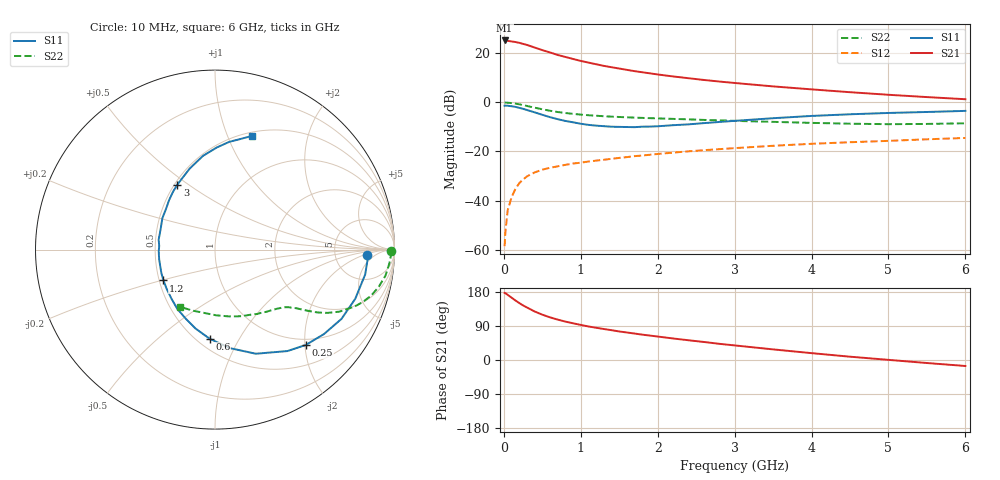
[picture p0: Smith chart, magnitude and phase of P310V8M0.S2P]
! SIEMENS Small Signal Semiconductors
! BFP181
! Si NPN RF Bipolar Junction Transistor in SOT143
! VCE = 10 V  IC = 8 mA
! Common Emitter S-Parameters:  March  1996
# GHz  S  MA  R  50
!  f  S11  S21  S12  S22
! GHz  MAG  ANG  MAG  ANG  MAG  ANG  MAG  ANG
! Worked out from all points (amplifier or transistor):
!   36 points, 10 MHz to 6 GHz, reference 50 ohm
!   highest |S21| = 25.1 dB at 10 MHz (marker M1)
!   |S21| within 3 dB of that: start of sweep to 413 MHz
!   unconditionally stable (mu >= 1): 1.558 GHz to end of sweep
!   at 250 MHz: K = 0.27, MSG = 27.5 dB, |S12| = -31.3 dB
!   at 1.4 GHz: K = 0.96, MSG = 18.6 dB, |S12| = -23.0 dB
!   at 6 GHz: K = 1.05, MAG = 6.5 dB, |S12| = -14.5 dB
!   S11 on the Smith chart (normalised r, x): 10 MHz: 12, -2; 250 MHz: 0.88, -2.02; 600 MHz: 0.58, -0.76; 1.2 GHz: 0.53, -0.20; 3 GHz: 0.52, +0.45; 6 GHz: 0.54, +1.23
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0.01  0.8483 -2.0  17.89 177.1  0.0012 73.8  0.9797 -0.6
0.02  0.852 -3.7  17.85 176.4  0.0023 85.7  0.9817 -1.6
0.05  0.8481 -9.4  17.55 171.9  0.0064 87.4  0.9749 -4.4
0.15  0.8036 -28.7  16.63 157.2  0.0174 73.2  0.9357 -12.8
0.2  0.7681 -37.8  16.03 150.4  0.0227 70.7  0.9072 -16.4
0.25  0.7336 -46.4  15.24 144.0  0.0271 66.5  0.8727 -19.6
0.3  0.6945 -54.5  14.53 138.6  0.0312 63.3  0.8386 -22.3
0.4  0.6231 -68.6  12.87 128.1  0.0376 57.9  0.7747 -26.5
0.5  0.5552 -81.4  11.38 119.6  0.0428 53.5  0.7183 -29.4
0.6  0.4971 -93.5  10.22 112.6  0.0467 51.4  0.6703 -31.5
0.7  0.4528 -103.9  9.089 106.6  0.05 49.7  0.6325 -32.9
0.8  0.4165 -113.4  8.278 101.3  0.0536 48.5  0.6032 -34.0
1.1  0.3468 -141.0  6.366 88.5  0.0626 46.1  0.5438 -36.6
1.2  0.3346 -149.1  5.886 85.1  0.0653 45.7  0.5314 -37.4
1.5  0.3157 -170.4  4.819 75.3  0.0741 45.1  0.5009 -39.9
1.8  0.3188 169.9  4.048 66.9  0.0828 43.9  0.4803 -43.1
2.2  0.3415 149.2  3.33 56.8  0.0948 42.1  0.4585 -47.9
3  0.4182 120.2  2.455 38.5  0.117 36.9  0.4181 -59.6
3.5  0.4732 107.3  2.092 28.0  0.1305 33.2  0.3993 -68.4
4.5  0.5686 89.1  1.595 8.7  0.1542 25.5  0.3664 -88.8
5.5  0.6332 76.9  1.27 -8.0  0.1768 18.8  0.3624 -110.5
6  0.6665 71.9  1.149 -15.8  0.1881 14.9  0.3735 -121.7
